PROGRAM MAIN
VAR CONSTANT
    cInitSource			: ST_MA_MultiArray_InitPars := ( eTypeCode := eMA_TypeCode_LREAL, nDims := 1, aDimSizes := [cBufferLength]);	
END_VAR
VAR                       
	(* Signal Generator *)
	nSample				: UDINT;  
	fbFunctionGeneratorf1	: FB_FunctionGenerator;
	fSetFrequencyf1		: LREAL := 230;		// Hz
	fSetAmplitudeA1		: LREAL := 8;		// peak amplitude of sin signal		
	fbFunctionGeneratorf2	: FB_FunctionGenerator;
	fSetFrequencyf2		: LREAL := 120;		// Hz
	fSetAmplitudeA2		: LREAL := 10;		// peak amplitude of sin signal		
	
	(* Source buffers *)	
	aBufferSignal1				: ARRAY[1..cOversamples] OF LREAL;  // signal part 1 
	aBufferSignal2				: ARRAY[1..cOversamples] OF LREAL;  // signal part 2
	aBuffer						: ARRAY[1..cOversamples] OF LREAL;  // aBufferSignal1 + aBufferSignal2
                  			
	fbSource			: FB_CMA_Source :=(	stInitPars := cInitSource, 
											nOwnID := eID_Source, 
											aDestIDs := [eID_EnvSpec]);		// Initialize source buffers
											
	(* Result buffers *)										
	aSpectrumResult		: ARRAY[1..cFFTResult] OF LREAL;					// local result variable <- from sink
    fbSink				: FB_CMA_Sink := (nOwnID := eID_Sink);				// Initialize sink buffers
	bCalculate			: BOOL;												// true if new result available
	
	(* error monitoring *)
	fbErrHist			: FB_HRErrHist;
	
END_VAR


(* signal generator - generate beat signal *)	
fbFunctionGeneratorf1(	fFrequency 	:= fSetFrequencyf1,
						fAmplitude 	:= fSetAmplitudeA1,
						eFunction 	:= E_FunctionType.Sine,
						aSignal		:= aBufferSignal1 );
fbFunctionGeneratorf2(	fFrequency 	:= fSetFrequencyf2,
						fAmplitude 	:= fSetAmplitudeA2,
						eFunction 	:= E_FunctionType.Sine,
						aSignal		:= aBufferSignal2 );	
						
FOR nSample := 1 TO cOversamples DO
	aBuffer[nSample] := aBufferSignal1[nSample]+aBufferSignal2[nSample];
END_FOR			
						
					

(* Call source to collect data *)
fbSource.Input1DStd( pDataIn 			:= ADR(aBuffer),
					  nDataInSize 		:= SIZEOF(aBuffer), 
					  eElementType 		:= eMA_TypeCode_LREAL,
					  nOptionPars		:= cCMA_Option_MarkInterruption ); 
IF fbSource.bError THEN
	fbErrHist.AddError(bErr:=TRUE, hrErrCode:=fbSource.hrErrorCode, sErrSource:='MAIN.fbSource'); // error monitoring
	// ToDo: if error
END_IF


(* Push results to sink *)
fbSink.Output1DStd(	pDataOut 		:= ADR(aSpectrumResult), 
					nDataOutSize 	:= SIZEOF(aSpectrumResult), 
					eElementType 	:= eMA_TypeCode_LREAL, 
					nOptionPars		:= 0,
					bNewResult		=> bCalculate );
IF fbSink.bError THEN
	fbErrHist.AddError(bErr:=TRUE, hrErrCode:=fbSink.hrErrorCode, sErrSource:='MAIN.fbSink'); // error monitoring
	// ToDo: if error
END_IF

END_PROGRAM
